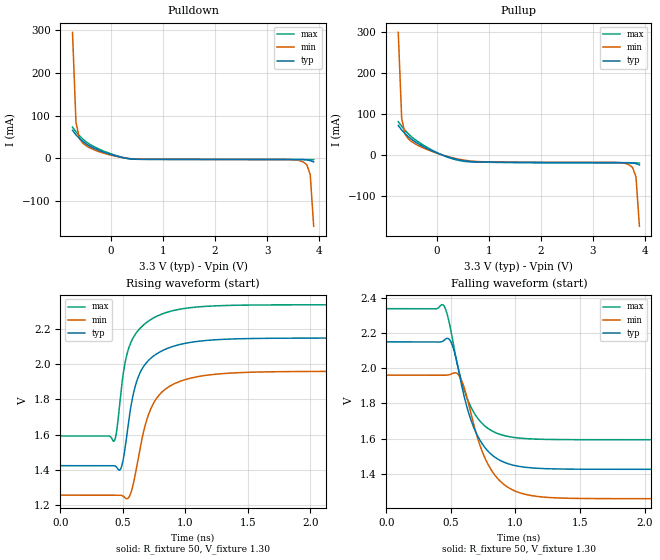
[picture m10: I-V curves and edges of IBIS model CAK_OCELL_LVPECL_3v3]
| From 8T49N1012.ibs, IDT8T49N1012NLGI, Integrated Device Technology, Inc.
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[Model] CAK_OCELL_LVPECL_3v3
Model_type   Output_ECL
Polarity   Non-Inverting
|   typ   min   max
C_comp   2pF   1.5pF   2.5pF
Vmeas= 1.865V
Rref = 50
Cref = 0
Vref = 1.3V
|   typ   min   max
[Voltage range]   3.3V   3.135V   3.465V
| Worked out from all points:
|   rising waveform, R_fixture 50, V_fixture 1.30: 20-80 % time 157ps typ, 178ps min, 150ps max; typ from 1.43 V to 2.15 V
|   falling waveform, R_fixture 50, V_fixture 1.30: 20-80 % time 188ps typ, 204ps min, 176ps max; typ from 2.15 V to 1.43 V
[Pulldown]
|Voltage   I (typ)   I (min)   I (max)
|Note, modeling breaks down at 250mA and above.  This is well beyond the functional   |
|operating range of the device.  Should this scenario occur, catastrophic failure and   |
|possible damage to the device and/or board is of higher concern than the I-V curve   |
|behavior.  The IBIS checker will flag currents in excess of 10A with warnings.  Lines   |
|with currents in excess of 0.35 A have been commented out.  The points still remain|
|available to the user if the user desires to use them.   |
|-2.84000e+00   3.76440e+01   3.02308e+01   4.60540e+01
|-2.38000e+00   2.88435e+01   2.36299e+01   3.48161e+01
|-1.92000e+00   2.00540e+01   1.70376e+01   2.35884e+01
|-1.46000e+00   1.12743e+01   1.04552e+01   1.23696e+01
|-1.00000e+00   2.50431e+00   3.88257e+00   1.16179e+00
|-9.99000e-01   2.48526e+00   3.86829e+00   1.13744e+00
|-9.32920e-01   1.22622e+00   2.92477e+00   1.70475e-01
|-8.66839e-01   2.57458e-01   1.98131e+00   9.45729e-02
|-8.00759e-01   8.77040e-02   1.03748e+00   8.32993e-02
-734.7mV  65.32mA    294.4mA    72.75mA
-668.6mV  54.93mA    84.39mA    62.14mA
-602.5mV  46.63mA    46.31mA    52.84mA
-536.4mV  39.56mA    35.36mA    44.92mA
-404.3mV  28.59mA    24.6mA     32.91mA
-140mV    14.59mA    12.2mA     17.09mA
388.7mV   -1.267mA   -923.5uA   -1.545mA
3.362V    -2.675mA   -2.655mA   -2.754mA
3.627V    -2.747mA   -5.58mA    -2.798mA
3.759V    -3.616mA   -14.88mA   -2.826mA
3.825V    -5.29mA    -37.77mA   -2.854mA
3.891V    -8.172mA   -158.7mA   -2.994mA
| 3.95703e+00   -1.21872e-02   -6.24127e-01   -3.64468e-03
| 4.02311e+00   -1.73234e-02   -1.17409e+00   -5.56365e-03
| 4.08920e+00   -2.56399e-02   -1.72433e+00   -9.14634e-03
| 4.15528e+00   -6.58984e-02   -2.27477e+00   -1.41884e-02
| 4.22136e+00   -4.33603e-01   -2.82537e+00   -2.02379e-02
| 4.28744e+00   -1.16649e+00   -3.37610e+00   -2.63820e-02
| 4.35352e+00   -1.90033e+00   -3.92693e+00   -3.48731e-02
| 4.41960e+00   -2.63437e+00   -4.47786e+00   -1.05263e-01
| 4.48568e+00   -3.36863e+00   -5.02887e+00   -8.14100e-01
| 4.55176e+00   -4.10310e+00   -5.57997e+00   -1.75185e+00
| 4.61784e+00   -4.83774e+00   -6.13115e+00   -2.68972e+00
| 4.68392e+00   -5.57255e+00   -6.68240e+00   -3.62770e+00
| 4.75000e+00   -6.30748e+00   -7.23372e+00   -4.56577e+00
| 4.75100e+00   -6.31860e+00   -7.24206e+00   -4.57997e+00
| 5.12080e+00   -1.04331e+01   -1.03286e+01   -9.83220e+00
| 5.49060e+00   -1.45495e+01   -1.34167e+01   -1.50881e+01
| 5.86040e+00   -1.86669e+01   -1.65062e+01   -2.03453e+01
| 6.23020e+00   -2.27853e+01   -1.95968e+01   -2.56032e+01
| 6.60000e+00   -2.69043e+01   -2.26884e+01   -3.08617e+01
[Pullup]
|Voltage   I (typ)   I (min)   I (max)
|Note, modeling breaks down at 250mA and above.  This is well beyond the functional   |
|operating range of the device.  Should this scenario occur, catastrophic failure and   |
|possible damage to the device and/or board is of higher concern than the I-V curve   |
|behavior.  The IBIS checker will flag currents in excess of 10A with warnings.  Lines   |
|with currents in excess of 0.35 A have been commented out.  The points still remain|
|available to the user if the user desires to use them.   |
|-2.84000e+00   3.76862e+01   3.02716e+01   4.60978e+01
|-2.38000e+00   2.88786e+01   2.36648e+01   3.48500e+01
|-1.92000e+00   2.00790e+01   1.70646e+01   2.36154e+01
|-1.46000e+00   1.12922e+01   1.04719e+01   1.23907e+01
|-1.00000e+00   2.51546e+00   3.89145e+00   1.17512e+00
|-9.99000e-01   2.49639e+00   3.87716e+00   1.15075e+00
|-9.32920e-01   1.23632e+00   2.93273e+00   1.82639e-01
|-8.66839e-01   2.66526e-01   1.98837e+00   1.05602e-01
|-8.00759e-01   9.57773e-02   1.04368e+00   9.32248e-02
-734.7mV  72.61mA    299.9mA    81.79mA
-668.6mV  61.59mA    89.42mA    70.45mA
-602.5mV  52.64mA    50.83mA    60.36mA
-536.4mV  44.82mA    39.32mA    51.52mA
-338.2mV  26.99mA    22.7mA     31.57mA
-7.793mV  6.385mA    5.56mA     7.349mA
520.9mV   -13.55mA   -11.76mA   -14.89mA
3.428V    -18.04mA   -17.54mA   -18.67mA
3.693V    -18.28mA   -23.28mA   -18.72mA
3.759V    -18.94mA   -29.63mA   -18.74mA
3.825V    -20.59mA   -52.53mA   -18.76mA
3.891V    -23.45mA   -173.4mA   -18.9mA
| 3.95703e+00   -2.74434e-02   -6.38902e-01   -1.95222e-02
| 4.02311e+00   -3.25618e-02   -1.18887e+00   -2.14116e-02
| 4.08920e+00   -4.08656e-02   -1.73912e+00   -2.49634e-02
| 4.15528e+00   -8.11177e-02   -2.28958e+00   -2.99791e-02
| 4.22136e+00   -4.48820e-01   -2.84019e+00   -3.60085e-02
| 4.28744e+00   -1.18171e+00   -3.39092e+00   -4.21403e-02
| 4.35352e+00   -1.91555e+00   -3.94175e+00   -5.06250e-02
| 4.41960e+00   -2.64962e+00   -4.49268e+00   -1.21010e-01
| 4.48568e+00   -3.38390e+00   -5.04370e+00   -8.29842e-01
| 4.55176e+00   -4.11838e+00   -5.59480e+00   -1.76758e+00
| 4.61784e+00   -4.85305e+00   -6.14598e+00   -2.70545e+00
| 4.68392e+00   -5.58787e+00   -6.69724e+00   -3.64342e+00
| 4.75000e+00   -6.32281e+00   -7.24856e+00   -4.58148e+00
| 4.75100e+00   -6.33394e+00   -7.25691e+00   -4.59568e+00
| 5.12080e+00   -1.04485e+01   -1.03434e+01   -9.84806e+00
| 5.49060e+00   -1.45649e+01   -1.34316e+01   -1.51041e+01
| 5.86040e+00   -1.86826e+01   -1.65213e+01   -2.03614e+01
| 6.23020e+00   -2.28013e+01   -1.96123e+01   -2.56197e+01
| 6.60000e+00   -2.69210e+01   -2.27045e+01   -3.08788e+01
[Ramp]
|   typ   min   max
dV/dt_r   0.449/0.155n   0.433/0.178n   0.464/0.146n
dV/dt_f   0.447/0.188n   0.429/0.205n   0.461/0.177n
R_load =   50.0000
[Rising Waveform]
R_fixture = 50
V_fixture = 1.30   | VCC_typ - 2V
V_fixture_max = 1.465   | VCC_max - 2V
V_fixture_min = 1.135   | VCC_min - 2V
C_fixture = 0.0p
| Time   typ   min   max
0s        1.425V     1.258V     1.593V
431.1ps   1.425V     1.258V     1.565V
488.9ps   1.418V     1.257V     1.871V
542.2ps   1.656V     1.241V     2.081V
591.1ps   1.854V     1.347V     2.16V
648.9ps   1.967V     1.564V     2.212V
742.2ps   2.045V     1.775V     2.261V
884.4ps   2.097V     1.879V     2.3V
1.476ns   2.145V     1.953V     2.335V
4ns       2.149V     1.96V      2.337V
[Falling Waveform]
R_fixture = 50
V_fixture = 1.30   | VCC_typ - 2V
V_fixture_max = 1.465   | VCC_max - 2V
V_fixture_min = 1.135   | VCC_min - 2V
C_fixture = 0.0p
| Time   typ   min   max
0s        2.15V      1.961V     2.339V
440ps     2.155V     1.96V      2.361V
497.8ps   2.154V     1.965V     2.226V
551.1ps   2.02V      1.969V     2.022V
626.7ps   1.775V     1.83V      1.828V
702.2ps   1.623V     1.615V     1.721V
795.6ps   1.522V     1.443V     1.654V
915.6ps   1.464V     1.336V     1.616V
1.342ns   1.427V     1.261V     1.594V
4ns       1.425V     1.258V     1.593V
